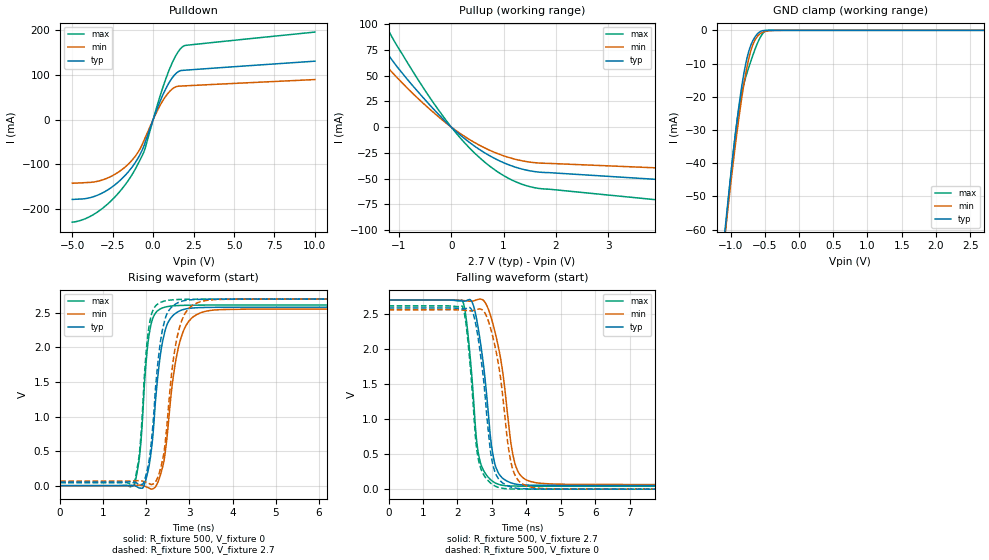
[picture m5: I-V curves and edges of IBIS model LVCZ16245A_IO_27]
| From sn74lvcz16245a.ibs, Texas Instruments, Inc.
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[Model]   LVCZ16245A_IO_27
Model_type  I/O
Vinl = 0.8
Vinh = 2
Enable   Active-Low
Vref =   0
Rref =   500
Cref =   30p
Vmeas =   1.35
| variable   typ   min   max
C_comp   3.57pF   3.07pF   4.16pF
| C_pullup   4.57pF   4.09pF   5.00pF
| C_pulldown   6.19pF   3.13pF   9.40pF
| C_tri-state   3.57pF   3.07pF   4.16pF
[Temperature Range]   40   100   -40
| Ambient temperature   25   85   -40
[Voltage range]   2.7   2.7   2.7
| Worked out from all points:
|   slope of the pulldown table from 0 to 0.405 V, typ, clamps not added: 10.5 ohm
|   slope of the pullup table from 0 to 0.405 V, typ, clamps not added: 23.8 ohm
|   GND clamp passes 1 mA (typ) near -0.60 V on its own axis
|   rising waveform, R_fixture 500, V_fixture 0: 20-80 % time 255ps typ, 318ps min, 186ps max; typ from 0 V to 2.58 V
|   falling waveform, R_fixture 500, V_fixture 2.7: 20-80 % time 357ps typ, 449ps min, 273ps max; typ from 2.7 V to 0.052 V
|   rising waveform, R_fixture 500, V_fixture 2.7: 20-80 % time 242ps typ, 292ps min, 179ps max; typ from 0.052 V to 2.7 V
|   falling waveform, R_fixture 500, V_fixture 0: 20-80 % time 340ps typ, 420ps min, 266ps max; typ from 2.59 V to 0 V
[GND Clamp]
| LVCZ16245A_IO_27
|   Voltage   I(typ)   I(min)   I(max)
-5V       -1.044A    -987.9mA   -1.125A
-1.08V    -59.89mA   -61.4mA    -61.3mA
-1.055V   -54.83mA   -56.68mA   -55.83mA
-980mV    -40.29mA   -43.08mA   -40.37mA
-915mV    -28.75mA   -32.11mA   -28.86mA
-860mV    -20.1mA    -23.65mA   -21.32mA
-805mV    -12.9mA    -16.19mA   -16.06mA
-755mV    -7.939mA   -10.55mA   -12.5mA
-700mV    -4.274mA   -5.894mA   -9.053mA
-590mV    -724.2uA   -1.404mA   -3.085mA
-470mV    -23.29uA   -236.4uA   -26.84uA
2.7V      1.12nA     59.79nA    439.8pA
[Pulldown]
| LVCZ16245A_IO_27
|   Voltage   I(typ)   I(min)   I(max)
-5V       -178.2mA   -142.1mA   -229.1mA
-4.075V   -175.7mA   -140.5mA   -219.4mA
-3.115V   -163.3mA   -134.5mA   -197.7mA
-2.17V    -139.8mA   -117.8mA   -165mA
-1.33V    -107.4mA   -91.7mA    -124.5mA
-885mV    -82.93mA   -70.03mA   -95.37mA
-535mV    -55.22mA   -44.07mA   -68.41mA
210mV     20.82mA    16.37mA    26.55mA
725mV     64.74mA    49.35mA    84.99mA
1.305V    98.85mA    71.39mA    136.2mA
1.815V    109.8mA    75.02mA    162.4mA
10V       130.4mA    89.33mA    195.3mA
[Pullup]
| LVCZ16245A_IO_27
|   Voltage   I(typ)   I(min)   I(max)
-5V       380mA      314.4mA    511.5mA
-1.96V    126.7mA    103.6mA    171.4mA
-1.8V     114.7mA    93.66mA    155.1mA
-1.58V    98.31mA    80.19mA    132.6mA
-1.265V   74.66mA    61.04mA    99.94mA
-890mV    49.44mA    40.43mA    66.89mA
-405mV    21.15mA    17.11mA    28.32mA
215mV     -9.551mA   -7.745mA   -12.99mA
870mV     -31.46mA   -25.38mA   -42.84mA
1.49V     -42.28mA   -33.85mA   -57.62mA
8.69V     -66.02mA   -49.55mA   -94.54mA
10V       -70.26mA   -52.32mA   -101.2mA
[Ramp]
| LVCZ16245A_IO_27
| variable   typ   min   max
dV/dt_r   1.57/2.69E-10   1.56/3.33E-10   1.58/1.96E-10
dV/dt_f   1.59/3.67E-10   1.59/4.60E-10   1.60/2.78E-10
R_load = 500
[Rising Waveform]
| LVCZ16245A_IO_27
R_fixture =   500
C_fixture =   0
L_fixture =   0
V_fixture =   0
V_fixture_min = 0
V_fixture_max = 0
|   Time   V(typ)   V(min)   V(max)
0s        102.4pV    3.006nV    7.332nV
1.72ns    565.6uV    3.006mV    8.633mV
1.92ns    -31.3mV    311.2uV    1.072V
2.015ns   150.6mV    -22.08mV   1.934V
2.125ns   562.9mV    -50.03mV   2.376V
2.35ns    1.994V     206.7mV    2.565V
2.62ns    2.463V     1.56V      2.602V
2.975ns   2.564V     2.372V     2.61V
3.775ns   2.582V     2.549V     2.614V
50ns      2.583V     2.555V     2.614V
[Falling Waveform]
| LVCZ16245A_IO_27
R_fixture =   500
C_fixture =   0
L_fixture =   0
V_fixture =   2.7
V_fixture_min = 2.7
V_fixture_max = 2.7
|   Time   V(typ)   V(min)   V(max)
0s        2.7V       2.7V       2.7V
2.135ns   2.686V     2.695V     2.699V
2.415ns   2.68V      2.683V     1.638V
2.555ns   2.436V     2.702V     711.4mV
2.68ns    2.058V     2.713V     361.5mV
3.03ns    498mV      2.363V     110.1mV
3.385ns   131.3mV    1.399V     50.36mV
3.755ns   66.96mV    259.3mV    43.97mV
4.64ns    53.85mV    76.66mV    41.75mV
50ns      52.01mV    65.51mV    41.19mV
[Rising Waveform]
| LVCZ16245A_IO_27
R_fixture =   500
C_fixture =   0
L_fixture =   0
V_fixture =   2.7
V_fixture_min = 2.7
V_fixture_max = 2.7
|   Time   V(typ)   V(min)   V(max)
0s        51.98mV    65.43mV    41.18mV
1.72ns    52.19mV    68.34mV    51.58mV
1.835ns   19.5mV     73.05mV    447.7mV
1.92ns    23.3mV     64.99mV    1.197V
2.12ns    661.2mV    16.14mV    2.482V
2.34ns    2.138V     276.1mV    2.655V
2.595ns   2.588V     1.676V     2.688V
2.92ns    2.682V     2.515V     2.697V
3.69ns    2.699V     2.695V     2.7V
50ns      2.7V       2.7V       2.7V
[Falling Waveform]
| LVCZ16245A_IO_27
R_fixture =   500
C_fixture =   0
L_fixture =   0
V_fixture =   0
V_fixture_min = 0
V_fixture_max = 0
|   Time   V(typ)   V(min)   V(max)
0s        2.587V     2.561V     2.617V
2.135ns   2.575V     2.557V     2.615V
2.405ns   2.569V     2.546V     1.561V
2.545ns   2.324V     2.564V     640.8mV
2.665ns   1.943V     2.571V     317.9mV
3ns       421.6mV    2.232V     73.04mV
3.355ns   76.12mV    1.151V     9.389mV
3.675ns   16.54mV    197.3mV    2.81mV
4.38ns    2.22mV     12.95mV    735.2uV
50ns      29.81uV    75.85uV    12.72uV
